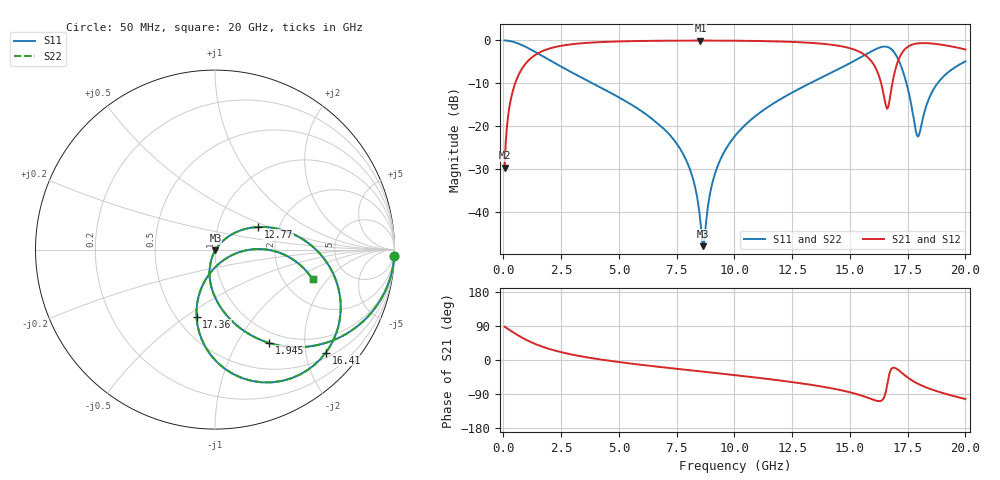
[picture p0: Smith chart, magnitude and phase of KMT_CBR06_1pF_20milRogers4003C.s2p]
! Data measured by Modelithics Inc. support@modelithics.com 813-866-6335
! KEMET CBR0603 1pF, Pad Width= 0.851mm, Pad Length= 0.64mm, Pad Gap= 0.62mm, 20mil Rogers 4003C substrate Data, January 2022
# hz S ma R 50
! 2 Port Network Data from SP1.SP block
! freq  magS11  angS11  magS21  angS21  magS12  angS12  magS22  angS22
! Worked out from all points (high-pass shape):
!   401 points, 50 MHz to 20 GHz, reference 50 ohm
!   highest |S21| = -0.04 dB at 8.529 GHz (marker M1); lowest = -29.7 dB at 50 MHz (marker M2)
!   |S21| within 3 dB of the highest: 1.483 GHz to 15.55 GHz (14.07 GHz wide, 165 % of centre); 17.24 GHz to end of sweep
!   lowest |S11| = -47.9 dB at 8.629 GHz (marker M3), VSWR 1.01, Z = 50.3 - j0.306 ohm
!   |S11| at or under -10 dB: 3.861 GHz to 13.26 GHz (9.403 GHz wide, 110 % of centre); 17.45 GHz to 18.79 GHz (1.342 GHz wide, 7.41 % of centre)
!   |S22| runs from -47.9 to 0.0 dB; largest |S21 - S12| = 0
!   S11 on the Smith chart (normalised r, x): 50 MHz: 1, -56; 1.945 GHz: 0.84, -1.37; 12.77 GHz: 1.56, +0.42; 16.41 GHz: 0.61, -2.41; 17.36 GHz: 0.63, -0.55; 20 GHz: 2.88, -1.41
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5e7  0.9995 -2.1  0.03286 87.9  0.03286 87.9  0.9995 -2.1
2.99375e8  0.981 -12.2  0.1933 77.7  0.1933 77.7  0.981 -12.2
5.98625e8  0.9298 -23.7  0.3673 66.2  0.3673 66.2  0.9298 -23.7
1.94525e9  0.6009 -59.9  0.7977 29.9  0.7977 29.9  0.6009 -59.9
3.391625e9  0.3681 -80.3  0.9275 9.4  0.9275 9.4  0.3681 -80.3
6.73325e9  0.1041 -105.7  0.9899 -18.1  0.9899 -18.1  0.1041 -105.7
7.980125e9  0.03663 -110.7  0.9954 -26.4  0.9954 -26.4  0.03663 -110.7
8.32925e9  0.01791 -106.7  0.9958 -28.7  0.9958 -28.7  0.01791 -106.7
8.52875e9  0.007692 -90.6  0.9959 -30.0  0.9959 -30.0  0.007692 -90.6
8.6285e9  0.004015 -49.3  0.9959 -30.7  0.9959 -30.7  0.004015 -49.3
9.177125e9  0.02909 47.8  0.9952 -34.3  0.9952 -34.3  0.02909 47.8
1.0025e10  0.07719 46.7  0.9922 -40.0  0.9922 -40.0  0.07719 46.7
1.276812e10  0.27 27.7  0.9544 -60.6  0.9544 -60.6  0.27 27.7
1.336662e10  0.3265 22.3  0.9348 -66.0  0.9348 -66.0  0.3265 22.3
1.531175e10  0.6026 -4.0  0.7596 -90.3  0.7596 -90.3  0.6026 -4.0
1.601e10  0.765 -23.7  0.5349 -104.8  0.5349 -104.8  0.765 -23.7
1.6409e10  0.8431 -42.9  0.2735 -105.4  0.2735 -105.4  0.8431 -42.9
1.670825e10  0.8215 -62.9  0.1948 -36.3  0.1948 -36.3  0.8215 -62.9
1.735662e10  0.3881 -105.4  0.7774 -39.2  0.7774 -39.2  0.3881 -105.4
1.795512e10  0.07584 -49.8  0.9254 -62.9  0.9254 -62.9  0.07584 -49.8
1.870325e10  0.2925 -0.1  0.9114 -81.2  0.9114 -81.2  0.2925 -0.1
2e10  0.569 -16.9  0.7846 -103.1  0.7846 -103.1  0.569 -16.9
